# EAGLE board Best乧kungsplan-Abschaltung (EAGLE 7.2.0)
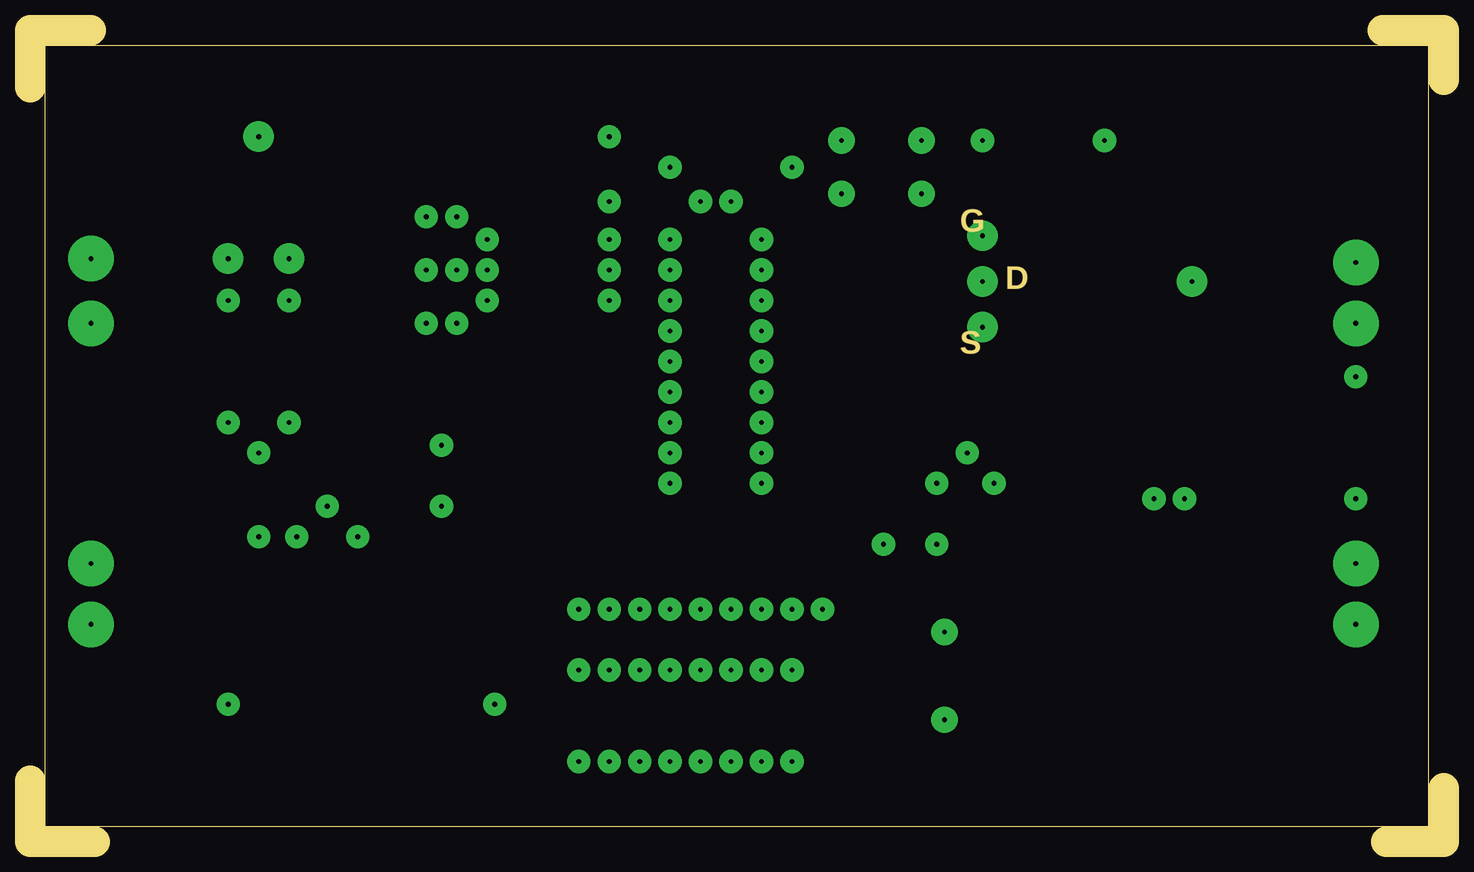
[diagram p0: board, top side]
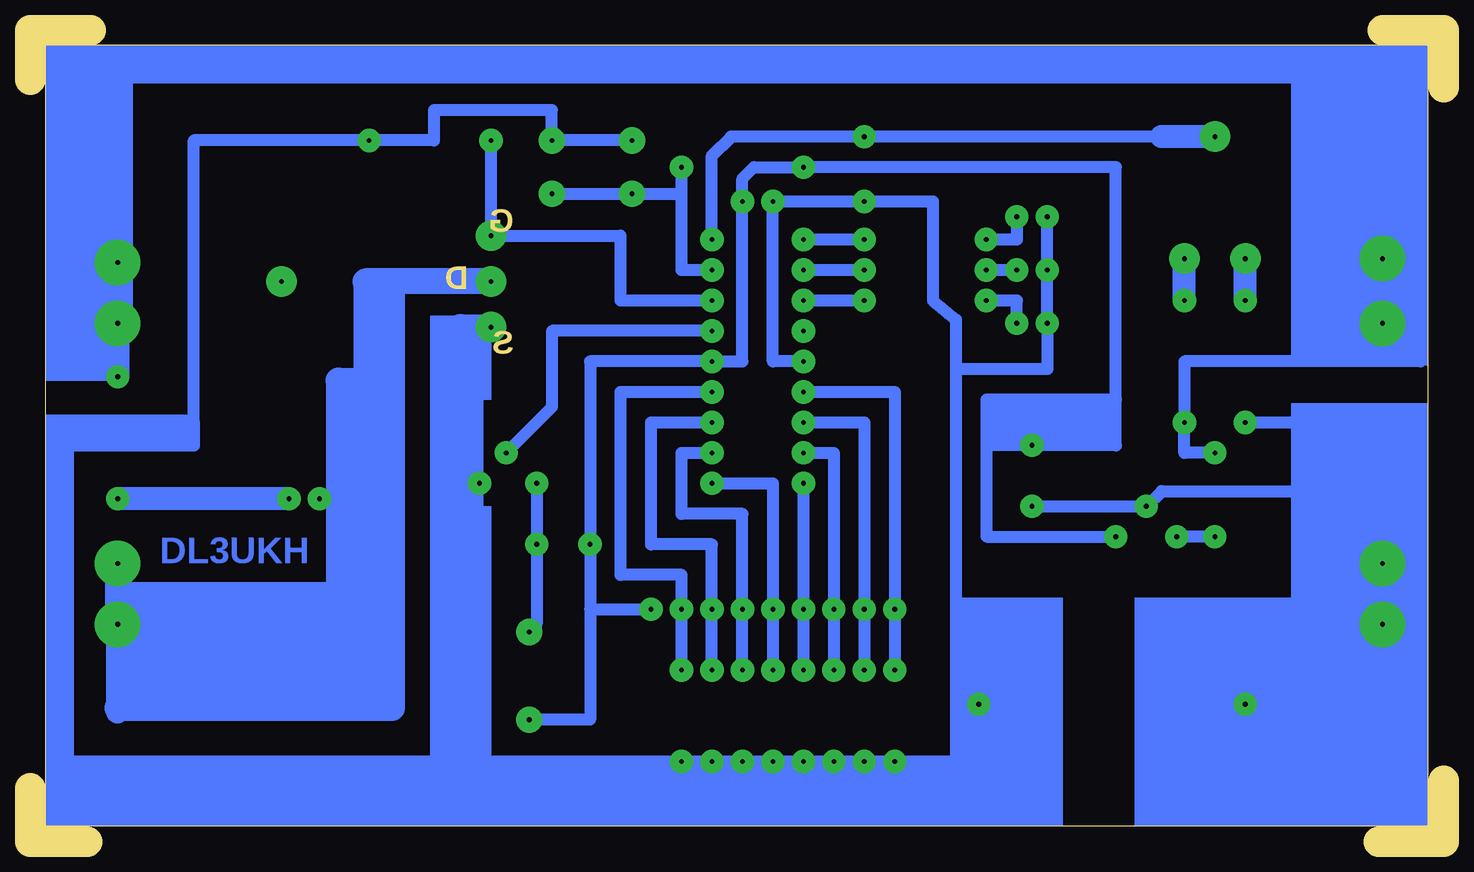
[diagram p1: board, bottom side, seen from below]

Size 117.79 x 67.63 mm. Coordinates in mm from the lower left corner, seen from the top.
Outline: 5.4,0 0.32,0
Outline: 0,0 0,5.08
Outline: 113.03,0 117.79,0 117.79,4.45
Outline: 5.08,67.63 0,67.63 0,62.87
Outline: 117.79,63.5 117.79,67.63
Outline: 112.71,67.63 117.47,67.63
Outline: 1.27,1.27 116.52,1.27 116.52,66.36 1.27,66.36 1.27,1.27
Copper layers (1*16): Top 0.035mm / dielectric 1.5mm / Bottom 0.035mm
Design rules "default": minimum track width 10mil, minimum drill 24mil, track to track 8mil, track to pad 8mil, pad to pad 8mil, via to via 8mil, smd to smd 8mil, copper to edge 40mil, drill to drill 8mil, minimum pad ring 10mil, minimum via ring 8mil, stop-mask expansion 4mil, vias tented up to drill 0mil, thermal gap 10mil

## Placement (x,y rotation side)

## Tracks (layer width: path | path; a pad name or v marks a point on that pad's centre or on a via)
S$1  (via drill 0.4 pad 1.93)
  Bottom 1.016: v19.05,25.4 v22.22,25.4
S$2  (via drill 0.4 pad 1.93, 0.4 pad 2.54)
  Bottom 1.016: v93.66,28.57 92.08,28.57
  Bottom 2.184: 92.08,11.11 92.08,28.57 92.08,38.42 87.63,38.42 87.63,46.67 | v79.38,46.67 87.63,46.67 | 87.63,46.67 89.85,46.67
S$3  (via drill 0.4 pad 2.18)
  other vias: 67.63,53.98
S$4  (via drill 0.4 pad 1.93)
  other vias: 53.34,42.55
S$5  (via drill 0.4 pad 1.93, 0.4 pad 2.18)
  Bottom 1.016: 27.3,36.83 27.3,33.02 38.1,33.02 | 27.3,36.83 27.3,56.2 v53.34,56.2 57.47,56.2 58.42,55.25 v58.42,53.34 58.42,40.01 v60.96,40.01 71.12,40.01 v71.12,24.77 71.12,19.37 | 38.1,33.02 38.1,32.38 38.1,25.4 v27.3,25.4 | 71.12,19.37 v66.04,19.37 | 71.12,19.37 71.12,10.16 v76.2,10.16 | 27.3,36.83 38.1,36.83 38.1,33.02
S$6  (via drill 0.4 pad 1.93, 0.4 pad 3.81)
  Bottom 1.016: 5.08,61.6 v5.08,48.58 v5.08,43.18 1.91,40.01 21.59,40.01 v21.59,34.93 21.59,32.38 v19.05,32.38
S$7  (via drill 0.4 pad 1.93)
  Bottom 1.016: v60.96,42.55 74.3,42.55 74.3,36.2 v78.1,32.38
S$8  (via drill 0.4 pad 1.93)
  other vias: 96.2,28.57
S$9  (via drill 0.4 pad 2.54)
  other vias: 96.84,46.67
S$11  (via drill 0.4 pad 1.93)
  other vias: 16.51,11.43
S$12  (via drill 0.4 pad 2.18)
  other vias: 74.3,58.42
S$13  (via drill 0.4 pad 1.93)
  Bottom 1.016: v80.33,29.84 81.6,29.84
S$14  (via drill 0.4 pad 1.93)
  Bottom 1.016: v53.34,37.47 45.72,37.47 v45.72,19.37 v45.72,14.29
S$15  (via drill 0.4 pad 1.93)
  Bottom 1.016: v53.34,34.93 48.26,34.93 v48.26,19.37 v48.26,14.29
S$16  (via drill 0.4 pad 1.93)
  Bottom 1.016: v53.34,32.38 50.8,32.38 v50.8,19.37 v50.8,14.29
S$17  (via drill 0.4 pad 1.93)
  Bottom 1.016: v53.34,29.84 v53.34,19.37 v53.34,14.29
S$18  (via drill 0.4 pad 1.93, 0.4 pad 3.81)
  Bottom 1.016: 110.49,61.6 v110.49,48.26 v110.49,43.18 110.49,42.86
  Bottom 1.93: 110.49,42.86 v110.49,38.74
  Bottom 2.184: v110.49,48.26 110.49,42.86
S$19  (via drill 0.4 pad 1.93, 0.4 pad 2.54)
  Bottom 1.016: v60.96,50.17 60.96,57.15 59.37,58.74 v48.26,58.74 23.5,58.74
  Bottom 1.93: v19.05,58.74 23.5,58.74
S$20  (via drill 0.4 pad 1.93)
  other vias: 34.29,33.02
S$21  (via drill 0.4 pad 3.81)
  Bottom 1.93: 110.49,10.79 110.49,11.11 v110.49,18.1
  Bottom 2.184: v110.49,23.18 v110.49,18.1 110.49,17.78 | 87.63,38.1 87.63,11.11 110.49,11.11
S$22  (via drill 0.4 pad 1.93)
  other vias: 38.74,11.43
S$23  (via drill 0.4 pad 1.93, 0.4 pad 2.18)
  Bottom 1.016: v60.96,47.62 63.5,47.62 63.5,53.98 | 63.5,53.98 v63.5,56.2 | v74.3,53.98 63.5,53.98
S$24  (via drill 0.4 pad 1.93, 0.4 pad 2.54)
  Bottom 1.016: v60.96,45.09 68.58,45.09 68.58,50.48 v79.38,50.48 v79.38,58.42
S$25  (via drill 0.4 pad 1.93)
  Bottom 1.016: v48.26,45.09 v53.34,45.09
S$26  (via drill 0.4 pad 1.93)
  Bottom 1.016: v60.96,29.84 55.88,29.84 v55.88,19.37 v55.88,14.29
S$27  (via drill 0.4 pad 1.93, 0.4 pad 2.18, 0.4 pad 2.54)
  Bottom 1.016: v33.02,52.07 v33.02,43.18 33.02,39.37 40.64,39.37 | v67.63,58.42 74.3,58.42 74.3,60.96 84.14,60.96 84.14,58.42 v89.53,58.42 104.14,58.42 104.14,34.93 | v53.34,40.01 55.88,40.01 v55.88,53.34 v48.26,53.34 42.55,53.34 42.55,45.09 40.64,43.5 40.64,39.37 | 40.64,39.37 40.64,6.67 81.91,6.67 114.62,6.67 114.62,34.93 104.14,34.93 | 114.94,33.02 104.14,33.02 104.14,34.93
  Bottom 2.184: v79.38,42.86 81.91,42.86 81.91,6.67
S$28  (via drill 0.4 pad 1.93)
  other vias: 45.72,6.67
S$29  (via drill 0.4 pad 1.93)
  other vias: 48.26,6.67
S$30  (via drill 0.4 pad 1.93)
  other vias: 50.8,6.67
S$31  (via drill 0.4 pad 1.93)
  other vias: 53.34,6.67
S$32  (via drill 0.4 pad 1.93)
  other vias: 55.88,6.67
S$33  (via drill 0.4 pad 1.93)
  other vias: 58.42,6.67
S$34  (via drill 0.4 pad 1.93)
  other vias: 60.96,6.67
S$35  (via drill 0.4 pad 1.93)
  other vias: 63.5,6.67
S$36  (via drill 0.4 pad 1.93, 0.4 pad 2.54)
  Bottom 1.93: v16.51,45.09 v16.51,48.58
S$37  (via drill 0.4 pad 1.93)
  Bottom 1.016: v48.26,47.62 v53.34,47.62
S$38  (via drill 0.4 pad 1.93)
  Bottom 1.016: v48.26,50.17 v53.34,50.17
S$39  (via drill 0.4 pad 1.93, 0.4 pad 2.54)
  Bottom 1.93: v21.59,45.09 v21.59,48.58
S$40  (via drill 0.4 pad 1.93)
  Bottom 1.016: v34.29,27.94 v24.77,27.94 23.5,29.21 11.75,29.21
S$42  (via drill 0.4 pad 1.93)
  Bottom 1.016: v35.56,52.07 35.56,50.17 v38.1,50.17
S$43  (via drill 0.4 pad 1.93)
  Bottom 1.016: v58.42,14.29 v58.42,19.37 58.42,27.3 63.5,27.3 63.5,32.38 v60.96,32.38
S$44  (via drill 0.4 pad 1.93)
  Bottom 1.016: v60.96,14.29 v60.96,19.37 60.96,24.77 66.04,24.77 66.04,34.93 v60.96,34.93
S$45  (via drill 0.4 pad 1.93)
  Bottom 1.016: v63.5,14.29 v63.5,19.37 63.5,22.22 68.58,22.22 68.58,37.47 v60.96,37.47
S$46  (via drill 0.4 pad 1.93, 0.4 pad 2.18)
  Bottom 1.016: v75.56,29.84 v75.56,24.77 75.56,18.1 v76.2,17.46
S$47  (via drill 0.4 pad 1.93, 0.4 pad 3.81)
  Bottom 1.016: v16.51,34.93 5.08,34.93 v5.08,23.18 v5.08,18.1 5.08,6.67
S$48  (via drill 0.4 pad 1.93)
  other vias: 33.02,47.62
S$49  (via drill 0.4 pad 1.93)
  Bottom 1.016: v35.56,47.62 v38.1,47.62
S$50  (via drill 0.4 pad 1.93)
  Bottom 1.93: 96.2,28.57 v110.49,28.57
S$52  (via drill 0.4 pad 1.93)
  Bottom 1.016: v35.56,43.18 35.56,45.09 v38.1,45.09
(copper drawn outside any net)
  shapes: Bottom area x22

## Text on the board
Bottom: DL3UKH
Pads: AUF BESTÜCKUNGS-SEITE GESEHEN
Dimension: G | S | D | G | D | S
tOrigins: IRF 1010 | PIC16F88 | 2N7000 | 1N4148 | 1 | Die Aussparung | Links oben ist | muß mit dem | immer PIN 1 | Bauelement | und dem Bestück- | ungsplan | Katode | Anode | µA78L05 | überein stimmen. | K | Widerstandsnetzwerk 8x10K | S | D | G | Alles mit 0,8mm vorbohren ! | Aufbohren: | Einstellreg. 250 1,2mm | Der Punkt auf dem Bauelement muß | Ausg. | Eing. | Taster 1,0mm | mit dem Punkt auf dem Bestückungs- | IRF1010 1,2mm | plan hier übereinstimmt. | Masse | Mosfet Befestigungsbohr... 3,2mm | Sicherungshalter 1,5mm | Summer 1,0mm | Aus- und Eingänge bei 1,2mm Cu-Draht | 2,0K | 10K | aufbohren mit 1,5mm | Siehe hierzu Fotos | Taster | K | 47n | 250 | gn | 470 | 47n | ge | K | 470 | Ausgang +Pol | rt | 470 | IRF 1010 | Eingang +Pol | K | 3,9K | 10K | LED rot/grün/gelb/blau | + | 2N7000 | PIC16F88 | bl | G | 1,2K | D | K | 47n | S | K | Eing. | 470/16 | 1N4148 | µA78L05 | 8x10K | Ausgang -Pol | K | 1 | 8 | Summer | wie | Eingang -Pol | Katode | 8fach DIP-Schalter | Sicherungshalter | + | Anode | immer an + Pol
